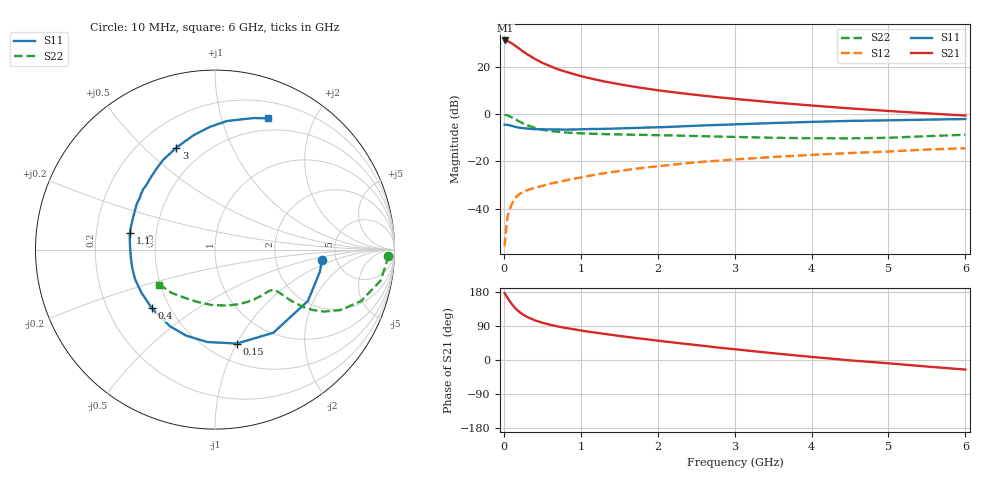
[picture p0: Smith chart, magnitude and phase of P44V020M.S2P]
! SIEMENS Small Signal Semiconductors
! BFP182
! Si NPN RF Bipolar Junction Transistor in SOT143
! VCE = 4 V  IC = 20 mA
! Common Emitter S-Parameters:  March  1996
# GHz  S  MA  R  50
!  f  S11  S21  S12  S22
! GHz  MAG  ANG  MAG  ANG  MAG  ANG  MAG  ANG
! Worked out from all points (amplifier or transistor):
!   36 points, 10 MHz to 6 GHz, reference 50 ohm
!   highest |S21| = 31.2 dB at 20 MHz (marker M1)
!   |S21| within 3 dB of that: start of sweep to 179.9 MHz
!   unconditionally stable (mu >= 1): 790.1 MHz to 5.363 GHz
!   at 250 MHz: K = 0.49, MSG = 29.8 dB, |S12| = -33.0 dB
!   at 1.4 GHz: K = 1.15, MAG = 16.6 dB, |S12| = -24.6 dB
!   at 6 GHz: K = 0.93, MSG = 6.9 dB, |S12| = -14.5 dB
!   S11 on the Smith chart (normalised r, x): 10 MHz: 3.85, -0.71; 150 MHz: 0.68, -1.00; 400 MHz: 0.40, -0.34; 1.1 GHz: 0.35, +0.08; 3 GHz: 0.35, +0.63; 6 GHz: 0.37, +1.42
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0.01  0.599 -5.7  36.27 176.3  0.0016 83.9  0.9652 -2.0
0.02  0.5972 -11.9  36.33 173.3  0.0026 83.0  0.9588 -4.2
0.05  0.5915 -28.9  35.27 163.2  0.0071 79.1  0.9387 -10.6
0.1  0.566 -55.0  31.69 148.5  0.0122 66.8  0.8627 -19.4
0.15  0.5373 -76.9  27.92 136.5  0.0168 60.7  0.7765 -25.7
0.2  0.5168 -94.9  24.34 127.1  0.0202 56.0  0.6992 -29.6
0.25  0.5054 -108.6  21.18 119.8  0.0223 52.8  0.6348 -31.9
0.3  0.4952 -120.4  18.67 114.1  0.0244 51.4  0.5835 -33.1
0.4  0.4803 -137.4  14.88 105.0  0.0276 50.5  0.5141 -33.9
0.5  0.4751 -150.0  12.21 98.3  0.0303 50.7  0.4702 -33.9
0.6  0.4749 -159.8  10.43 93.1  0.0337 51.4  0.4422 -33.8
0.7  0.4724 -167.7  8.955 88.6  0.0362 52.1  0.4232 -33.8
0.9  0.4726 179.8  7.117 81.5  0.0428 52.9  0.3992 -34.3
1.1  0.4831 169.2  5.853 74.7  0.0493 53.6  0.387 -35.8
1.3  0.4878 160.6  4.948 69.1  0.056 53.6  0.378 -37.8
1.6  0.5047 149.8  4.033 61.0  0.0656 52.7  0.3688 -41.7
2.2  0.5405 130.8  2.914 46.3  0.0853 49.3  0.3537 -51.6
3  0.6077 110.7  2.107 28.4  0.1099 42.8  0.3294 -68.3
3.5  0.6484 100.6  1.771 17.9  0.1235 38.2  0.3156 -80.6
4.5  0.7193 84.7  1.323 -1.0  0.1499 29.6  0.3071 -108.0
5.5  0.7647 73.5  1.04 -17.3  0.178 21.7  0.3415 -135.1
6  0.7874 68.1  0.935 -25.2  0.1893 16.8  0.3661 -147.9
